(* Logix 5000 AddOnInstructionDefinition export B256_SLEtoS; software revision 30.00 *)

ADD_ON_INSTRUCTION B256_SLEtoS   (* revision 1.0 20170916, vendor Kenneth A. Fischer *)
// Convert 256-bit little-endian string to a big-endian string
// Revision note:
// Rev1.0: 20170916 - Initial Release
VAR_IN_OUT
   In_S : STRING; {required}
   Out_S : STRING; {required}
END_VAR

ROUTINE Logic   (* ladder *)
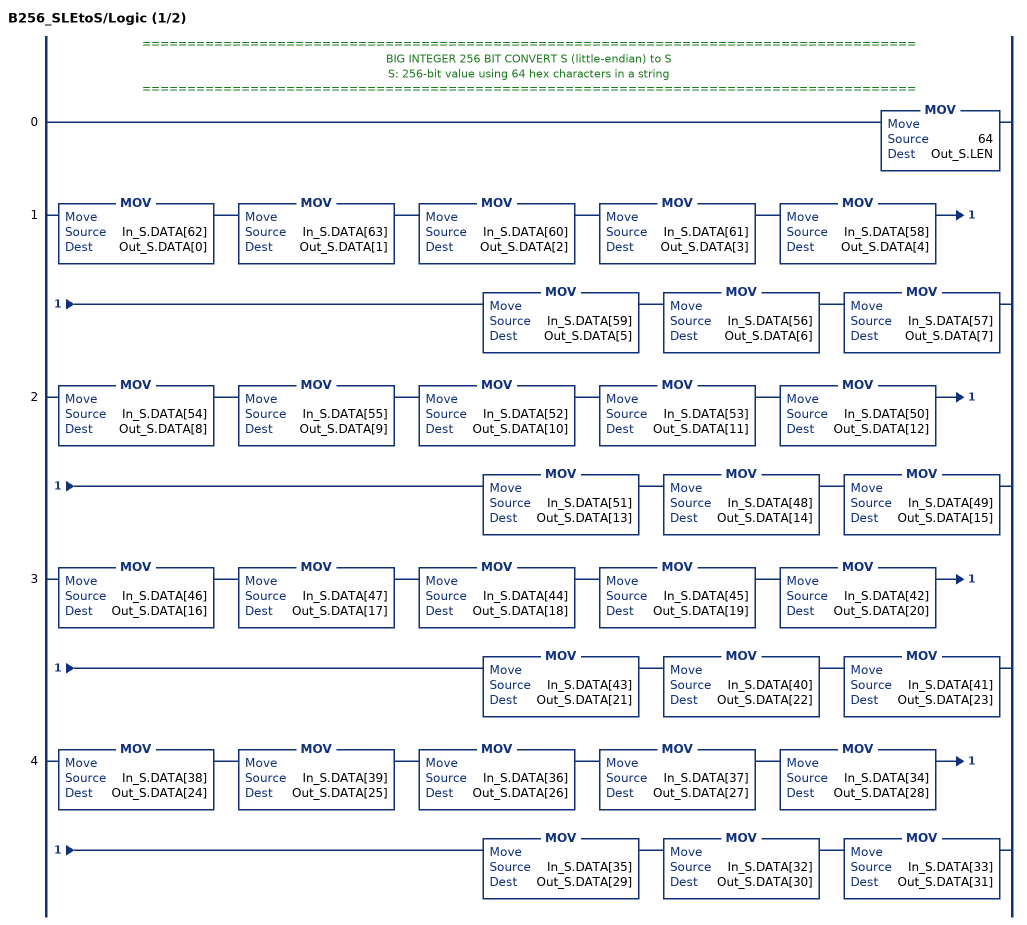
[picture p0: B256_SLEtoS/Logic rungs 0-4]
   // ======================================================================================
   // BIG INTEGER 256 BIT CONVERT S (little-endian) to S
   // S: 256-bit value using 64 hex characters in a string
   // ======================================================================================
   0: MOV(64,Out_S.LEN);
   1: MOV(In_S.DATA[62],Out_S.DATA[0])MOV(In_S.DATA[63],Out_S.DATA[1])MOV(In_S.DATA[60],Out_S.DATA[2])MOV(In_S.DATA[61],Out_S.DATA[3])MOV(In_S.DATA[58],Out_S.DATA[4])MOV(In_S.DATA[59],Out_S.DATA[5])MOV(In_S.DATA[56],Out_S.DATA[6])MOV(In_S.DATA[57],Out_S.DATA[7]);
   2: MOV(In_S.DATA[54],Out_S.DATA[8])MOV(In_S.DATA[55],Out_S.DATA[9])MOV(In_S.DATA[52],Out_S.DATA[10])MOV(In_S.DATA[53],Out_S.DATA[11])MOV(In_S.DATA[50],Out_S.DATA[12])MOV(In_S.DATA[51],Out_S.DATA[13])MOV(In_S.DATA[48],Out_S.DATA[14])MOV(In_S.DATA[49],Out_S.DATA[15]);
   3: MOV(In_S.DATA[46],Out_S.DATA[16])MOV(In_S.DATA[47],Out_S.DATA[17])MOV(In_S.DATA[44],Out_S.DATA[18])MOV(In_S.DATA[45],Out_S.DATA[19])MOV(In_S.DATA[42],Out_S.DATA[20])MOV(In_S.DATA[43],Out_S.DATA[21])MOV(In_S.DATA[40],Out_S.DATA[22])MOV(In_S.DATA[41],Out_S.DATA[23]);
   4: MOV(In_S.DATA[38],Out_S.DATA[24])MOV(In_S.DATA[39],Out_S.DATA[25])MOV(In_S.DATA[36],Out_S.DATA[26])MOV(In_S.DATA[37],Out_S.DATA[27])MOV(In_S.DATA[34],Out_S.DATA[28])MOV(In_S.DATA[35],Out_S.DATA[29])MOV(In_S.DATA[32],Out_S.DATA[30])MOV(In_S.DATA[33],Out_S.DATA[31]);
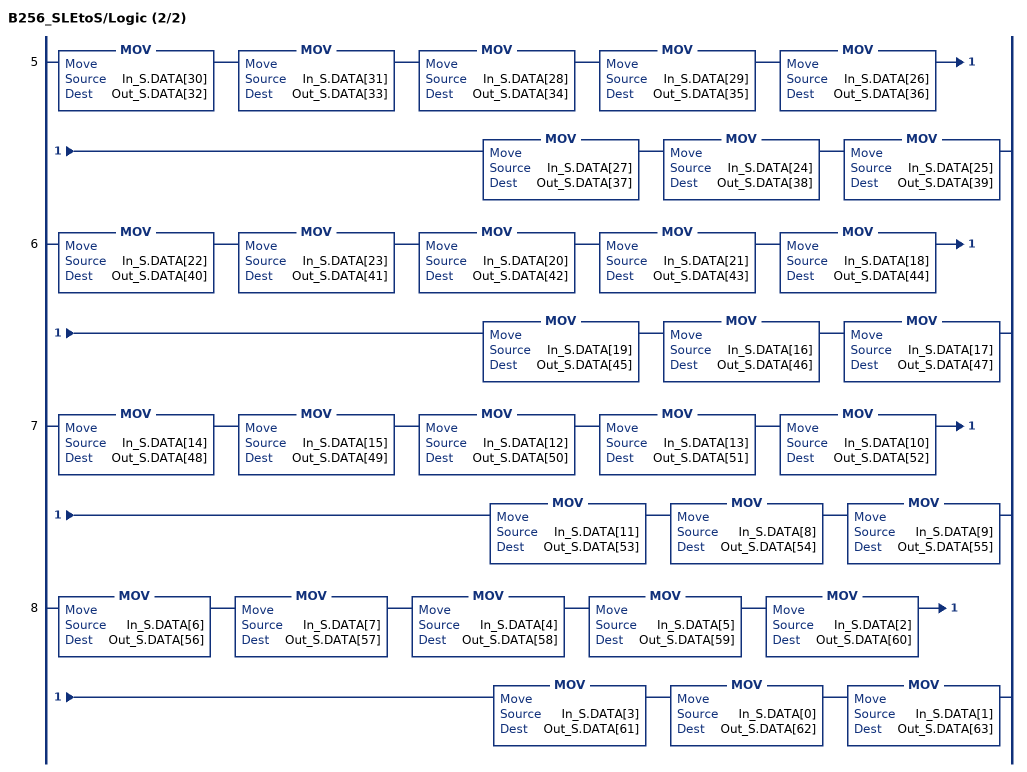
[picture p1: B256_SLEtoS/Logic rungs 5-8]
   5: MOV(In_S.DATA[30],Out_S.DATA[32])MOV(In_S.DATA[31],Out_S.DATA[33])MOV(In_S.DATA[28],Out_S.DATA[34])MOV(In_S.DATA[29],Out_S.DATA[35])MOV(In_S.DATA[26],Out_S.DATA[36])MOV(In_S.DATA[27],Out_S.DATA[37])MOV(In_S.DATA[24],Out_S.DATA[38])MOV(In_S.DATA[25],Out_S.DATA[39]);
   6: MOV(In_S.DATA[22],Out_S.DATA[40])MOV(In_S.DATA[23],Out_S.DATA[41])MOV(In_S.DATA[20],Out_S.DATA[42])MOV(In_S.DATA[21],Out_S.DATA[43])MOV(In_S.DATA[18],Out_S.DATA[44])MOV(In_S.DATA[19],Out_S.DATA[45])MOV(In_S.DATA[16],Out_S.DATA[46])MOV(In_S.DATA[17],Out_S.DATA[47]);
   7: MOV(In_S.DATA[14],Out_S.DATA[48])MOV(In_S.DATA[15],Out_S.DATA[49])MOV(In_S.DATA[12],Out_S.DATA[50])MOV(In_S.DATA[13],Out_S.DATA[51])MOV(In_S.DATA[10],Out_S.DATA[52])MOV(In_S.DATA[11],Out_S.DATA[53])MOV(In_S.DATA[8],Out_S.DATA[54])MOV(In_S.DATA[9],Out_S.DATA[55]);
   8: MOV(In_S.DATA[6],Out_S.DATA[56])MOV(In_S.DATA[7],Out_S.DATA[57])MOV(In_S.DATA[4],Out_S.DATA[58])MOV(In_S.DATA[5],Out_S.DATA[59])MOV(In_S.DATA[2],Out_S.DATA[60])MOV(In_S.DATA[3],Out_S.DATA[61])MOV(In_S.DATA[0],Out_S.DATA[62])MOV(In_S.DATA[1],Out_S.DATA[63]);
END_ROUTINE
END_ADD_ON_INSTRUCTION
